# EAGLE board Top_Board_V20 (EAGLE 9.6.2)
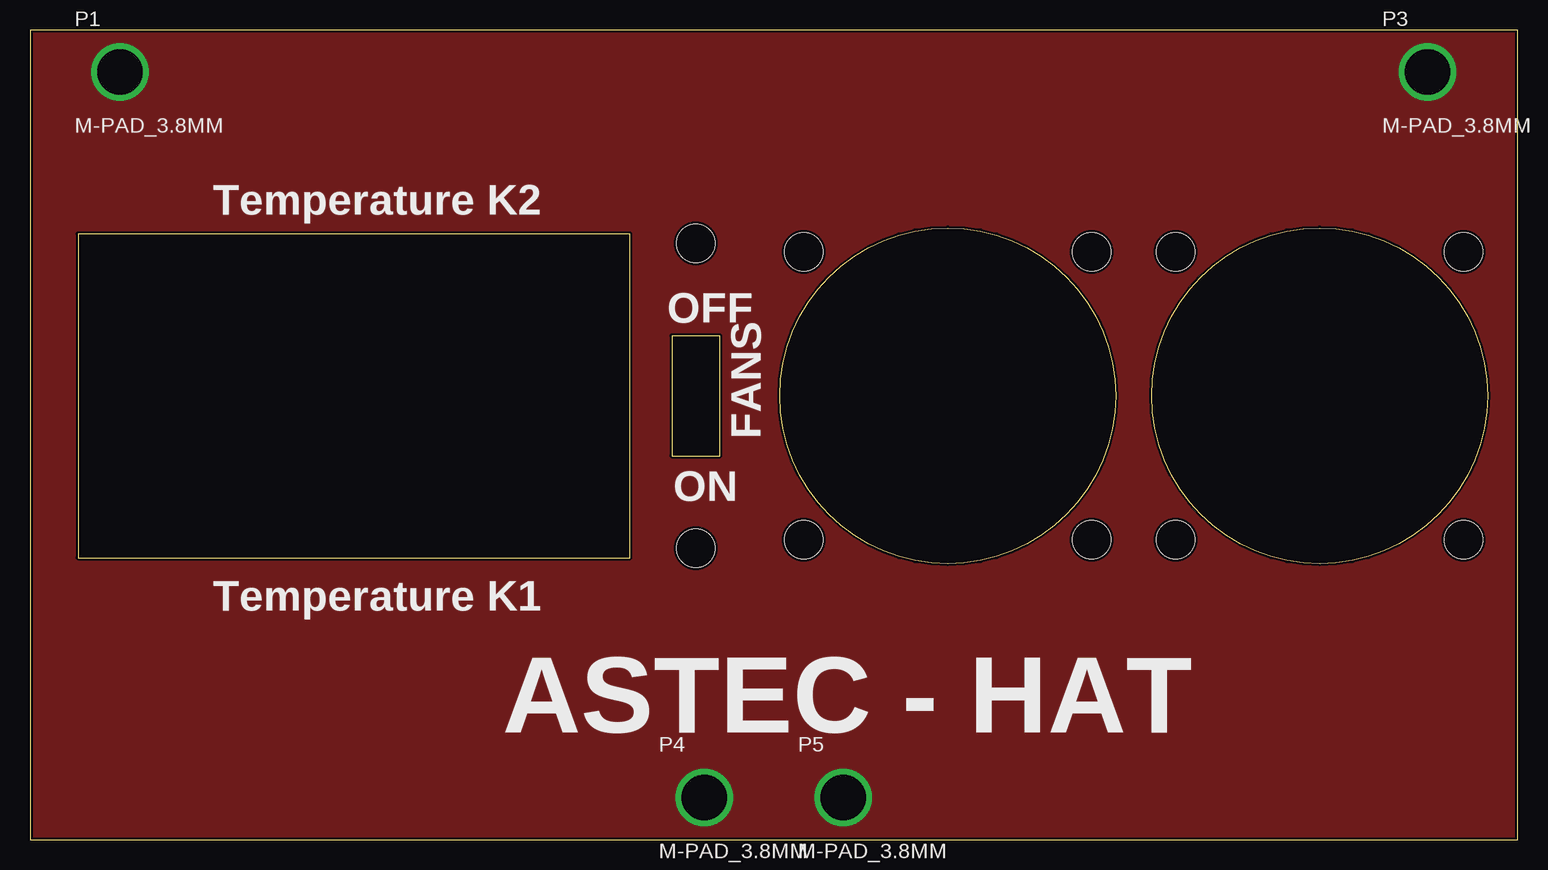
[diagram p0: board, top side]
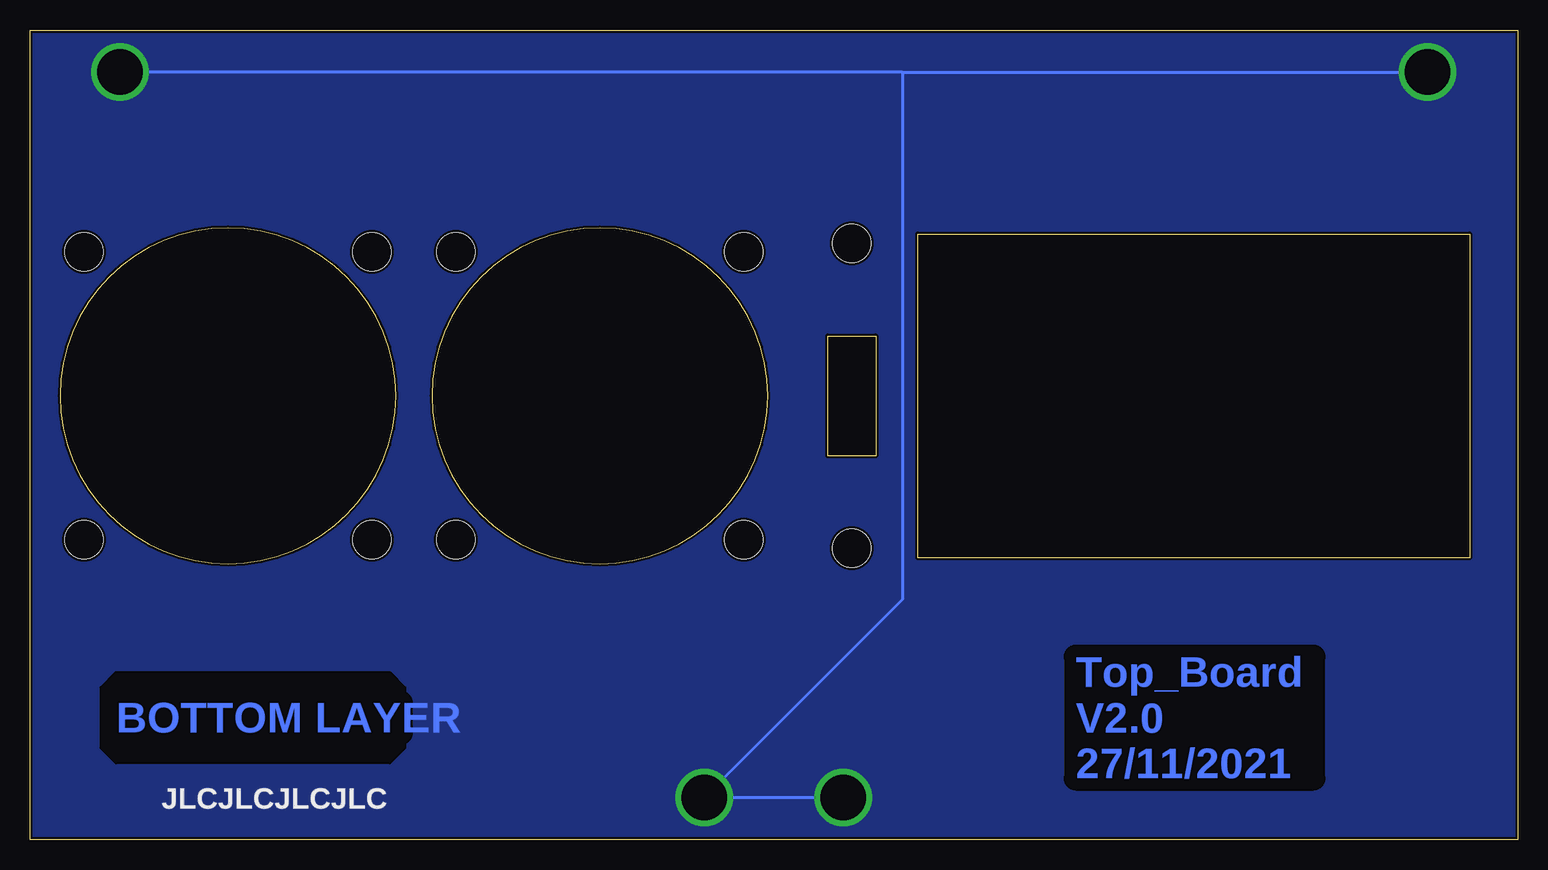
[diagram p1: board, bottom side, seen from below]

Size 124 x 67.5 mm. Coordinates in mm from the lower left corner, seen from the top.
Outline: 0,0 124,0 124,67.5 0,67.5 0,0
Outline: 4,23.5 50,23.5 50,50.5 4,50.5 4,23.5
Outline: 53.5,42 53.5,32 57.5,32 57.5,42 53.5,42
Outline: 62.5,37 arc-180 90.5,37 arc-180 62.5,37
Outline: 93.5,37 arc-180 121.5,37 arc-180 93.5,37
Copper layers (1*16): Top 0.035mm / dielectric 1.5mm / Bottom 0.035mm
Design rules "JLCPCB_2alyer": minimum track width 5mil, minimum drill 0.2mm, track to track 5mil, track to pad 0.2mm, pad to pad 0.2mm, via to via 0.2mm, smd to smd 5mil, copper to edge 0.2mm, drill to drill 0.5mm, minimum pad ring 0.13mm, minimum via ring 0.13mm, stop-mask expansion 0.05mm, vias tented up to drill 0mil, thermal gap 10mil
Net classes: 1 Versorgung: clearance 1 mm
Holes 3.2 mm at 55.5,49.7 55.5,24.3 64.5,25 88.5,25 95.5,25 119.5,25 119.5,49 95.5,49 88.5,49 64.5,49
bRestrict: 8 lines
Milling: 12 lines

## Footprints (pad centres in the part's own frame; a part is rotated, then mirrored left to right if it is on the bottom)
M-PAD_3.8MM = drill 3.8 pad 4.4: P$1 0,0

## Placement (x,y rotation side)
P1  M-PAD_3.8MM  [M-PAD_3.8MM]  7.5,64 0 top
P3  M-PAD_3.8MM  [M-PAD_3.8MM]  116.5,64 0 top
P4  M-PAD_3.8MM  [M-PAD_3.8MM]  56.2,3.5 0 top
P5  M-PAD_3.8MM  [M-PAD_3.8MM]  67.8,3.5 0 top

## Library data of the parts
P1 P3-P5 = Antec-Hood

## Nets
GND [Versorgung]: P1.P$1 P3.P$1 P4.P$1 P5.P$1

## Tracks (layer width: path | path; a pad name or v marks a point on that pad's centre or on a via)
GND
  Bottom 0.254: 51.29,64 P3.P$1 | P4.P$1 P5.P$1 51.29,20.01 51.29,64 | 51.29,64 P1.P$1
  pour Bottom (no thermals): -1.27,68.58 -1.27,-2.54 0,-3.81 127,-3.81 127,69.85 125.73,71.12 1.27,71.12
  pour Top (no thermals): -2.54,71.12 -2.54,-3.81 -1.27,-5.08 125.73,-5.08 127,-3.81 127,69.85 123.19,73.66 -1.27,73.66 -2.54,72.39

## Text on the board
Bottom: BOTTOM LAYER | Top_Board / V2.0 / 27/11/2021
tPlace: Temperature K2 | OFF | FANS | ON | Temperature K1 | ASTEC - HAT
bPlace: JLCJLCJLCJLC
